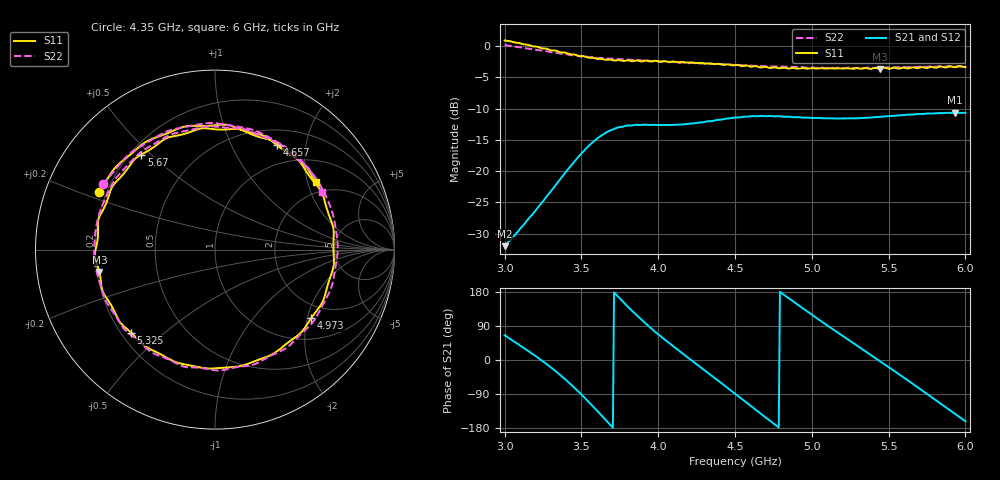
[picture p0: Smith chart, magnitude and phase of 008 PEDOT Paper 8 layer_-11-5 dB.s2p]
!  04/11/2025  19:50:17
! Ref Plane: 0.000 mm
# MHZ S MA R  50
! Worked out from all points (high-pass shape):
!   401 points, 3 GHz to 6 GHz, reference 50 ohm
!   highest |S21| = -10.67 dB at 5.933 GHz (marker M1); lowest = -32.0 dB at 3 GHz (marker M2)
!   |S21| within 3 dB of the highest: 3.672 GHz to end of sweep
!   lowest |S11| = -3.7 dB at 5.445 GHz (marker M3), VSWR 4.81, Z = 10.5 - j4.57 ohm
!   |S11| at or under -10 dB: nowhere
!   |S22| runs from -3.6 to 0.2 dB; largest |S21 - S12| = 0.0052
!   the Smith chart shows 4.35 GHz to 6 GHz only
!   S11 on the Smith chart (normalised r, x): 4.35 GHz: 0.17, +0.23; 4.657 GHz: 0.70, +1.51; 4.973 GHz: 1.57, -2.12; 5.325 GHz: 0.24, -0.39; 5.67 GHz: 0.24, +0.47; 6 GHz: 1.63, +2.27
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3000  1.106 -111.6  0.02518 65.2  0.02534 66.2  1.018 -115.8
3270  0.9524 -178.9  0.06213 -9.7  0.062 -8.8  0.9075 177.0
3390  0.8869 143.9  0.0957 -49.2  0.09614 -48.9  0.8642 139.1
3502.5  0.8298 102.1  0.1396 -92.1  0.1398 -91.9  0.8252 96.9
3607.5  0.7885 58.2  0.1843 -136.0  0.1847 -135.9  0.7993 53.3
3735  0.7698 1.8  0.223 168.6  0.2235 169.3  0.7843 -2.2
3870  0.7636 -52.9  0.2342 114.0  0.2361 114.8  0.7712 -56.4
4005  0.7492 -100.3  0.2337 66.4  0.2335 67.0  0.7518 -103.1
4170  0.7408 -152.2  0.2367 13.5  0.2372 13.8  0.7365 -154.9
4350  0.7212 153.8  0.2513 -42.0  0.2522 -41.2  0.7208 149.8
4500  0.7043 107.2  0.268 -89.1  0.2699 -88.5  0.7024 101.6
4657.5  0.6766 59.5  0.2755 -138.3  0.2763 -138.0  0.6928 50.4
4807.5  0.6681 12.7  0.2729 175.2  0.2733 176.0  0.6838 2.0
4972.5  0.6578 -35.4  0.2678 127.2  0.2677 127.8  0.6717 -47.4
5002.5  0.6653 -44.0  0.2659 118.8  0.2658 119.3  0.6759 -55.5
5167.5  0.6626 -91.1  0.2634 72.7  0.2635 73.1  0.6701 -101.7
5325  0.6573 -135.3  0.2657 29.8  0.2665 30.2  0.6685 -142.7
5445  0.6558 -169.1  0.2717 -3.3  0.2727 -2.6  0.6735 -175.2
5505  0.6562 174.1  0.2752 -19.9  0.2766 -19.1  0.674 168.4
5670  0.6696 127.8  0.2839 -66.6  0.2853 -65.7  0.6797 122.7
5932.5  0.6759 52.8  0.2927 -142.1  0.2946 -141.5  0.6814 47.6
6000  0.6785 33.7  0.2923 -161.6  0.2935 -161.2  0.6802 28.3
